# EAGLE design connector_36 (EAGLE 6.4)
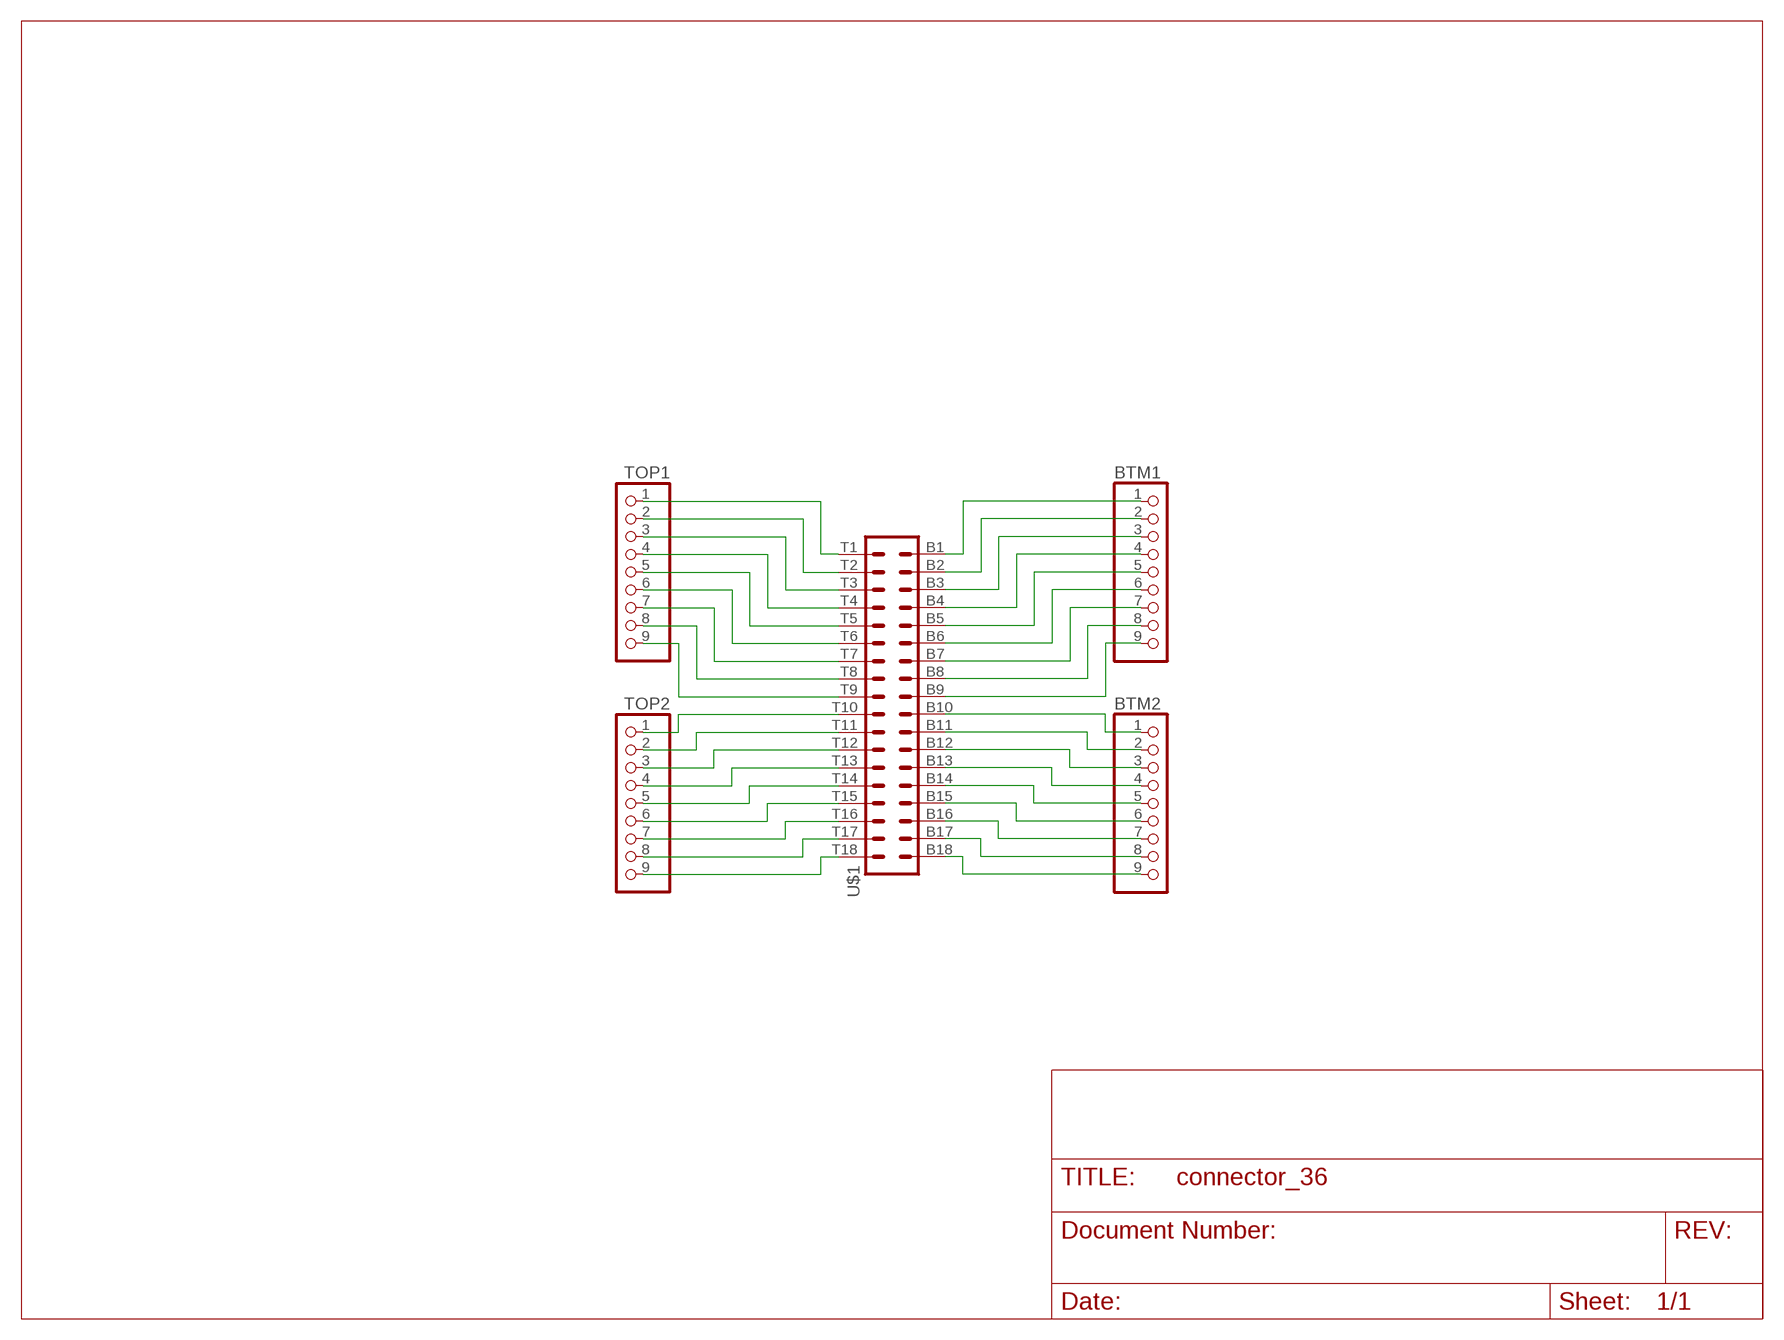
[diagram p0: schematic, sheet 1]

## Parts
BTM1  PINHD-1X9  [1X09]
BTM2  PINHD-1X9  [1X09]
TOP1  PINHD-1X9  [1X09]
TOP2  PINHD-1X9  [1X09]
U$1  OMNETICS_A79024-001  [OMNETICS_A79024-001]

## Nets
N$1: TOP1.1 U$1.T1
N$2: TOP1.2 U$1.T2
N$3: TOP1.3 U$1.T3
N$4: TOP1.4 U$1.T4
N$5: TOP1.5 U$1.T5
N$6: TOP1.6 U$1.T6
N$7: TOP1.7 U$1.T7
N$8: TOP1.8 U$1.T8
N$9: TOP1.9 U$1.T9
N$10: TOP2.1 U$1.T10
N$11: TOP2.2 U$1.T11
N$12: TOP2.3 U$1.T12
N$13: TOP2.4 U$1.T13
N$14: TOP2.5 U$1.T14
N$15: TOP2.6 U$1.T15
N$16: TOP2.7 U$1.T16
N$17: TOP2.8 U$1.T17
N$18: TOP2.9 U$1.T18
N$19: BTM1.1 U$1.B1
N$20: BTM1.2 U$1.B2
N$21: BTM1.3 U$1.B3
N$22: BTM1.4 U$1.B4
N$23: BTM1.5 U$1.B5
N$24: BTM1.6 U$1.B6
N$25: BTM1.7 U$1.B7
N$26: BTM1.8 U$1.B8
N$27: BTM1.9 U$1.B9
N$28: BTM2.1 U$1.B10
N$29: BTM2.2 U$1.B11
N$30: BTM2.3 U$1.B12
N$31: BTM2.4 U$1.B13
N$32: BTM2.5 U$1.B14
N$33: BTM2.6 U$1.B15
N$34: BTM2.7 U$1.B16
N$35: BTM2.8 U$1.B17
N$36: BTM2.9 U$1.B18

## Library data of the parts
BTM1 BTM2 TOP1 TOP2 = pinhead:PINHD-1X9: PIN HEADER
U$1 = omnetics_vic:OMNETICS_A79024-001

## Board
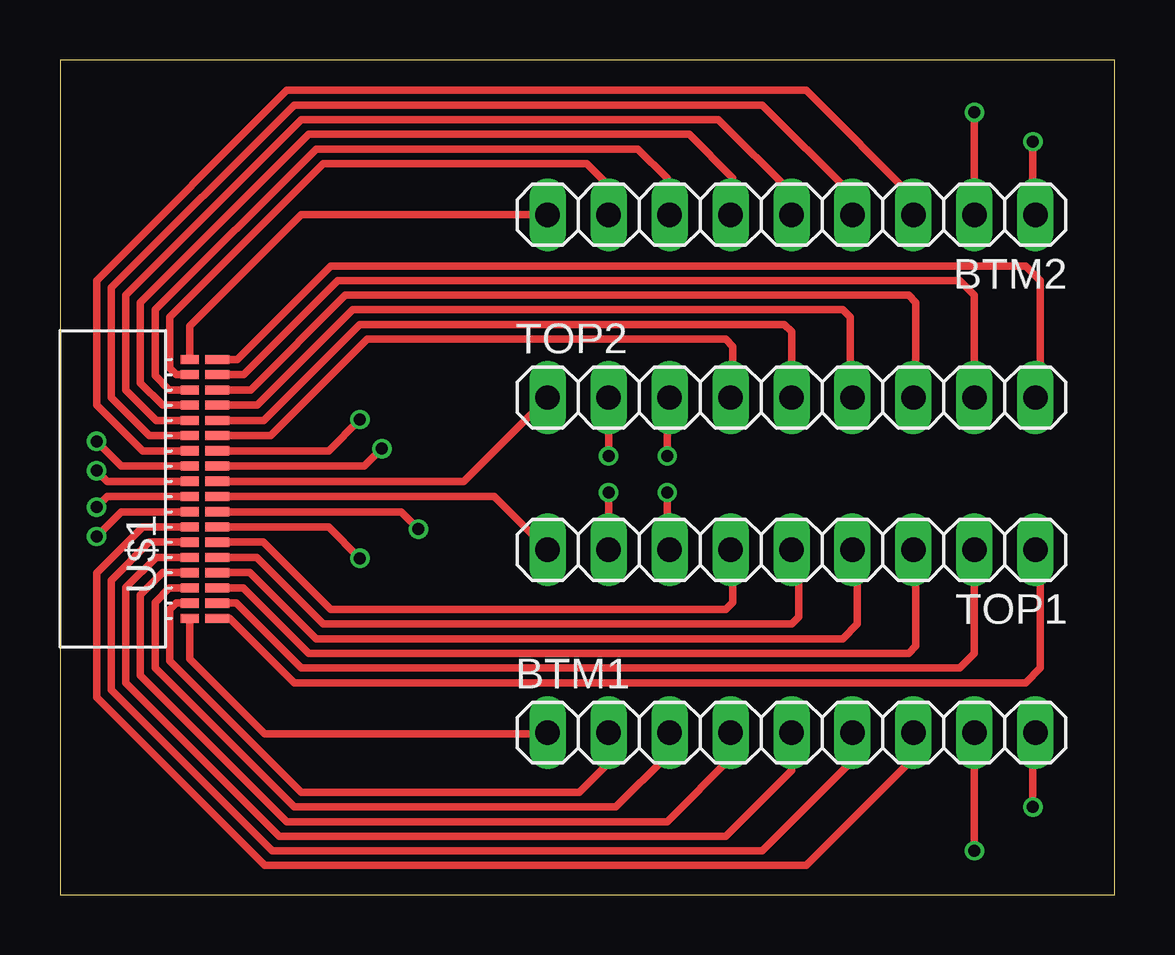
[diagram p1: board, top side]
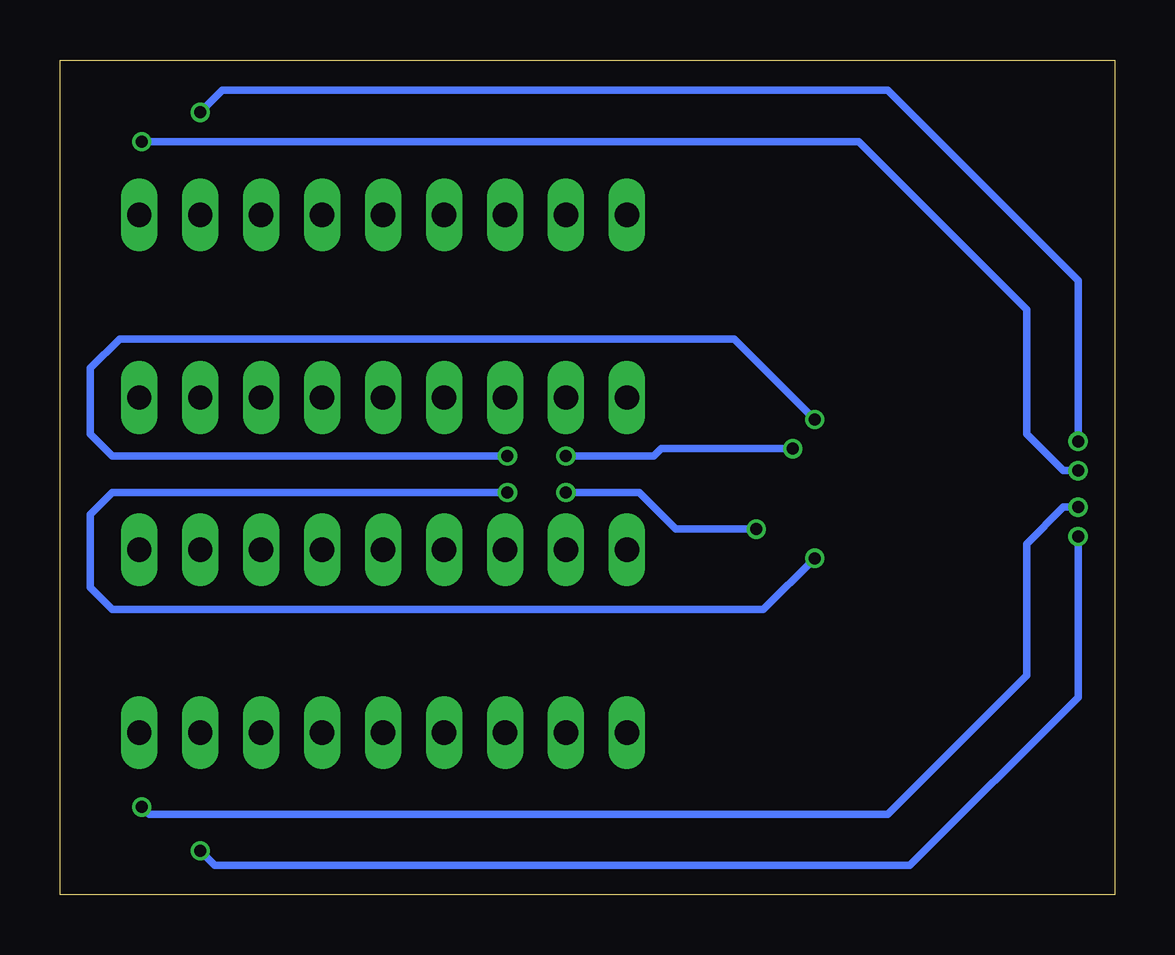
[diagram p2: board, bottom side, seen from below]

Size 43.94 x 34.8 mm. Coordinates in mm from the lower left corner, seen from the top.
Outline: 0,0 43.94,0 43.94,34.8 0,34.8 0,0
Copper layers (1*16): Top 0.035mm / dielectric 1.5mm / Bottom 0.035mm
Design rules "default *": minimum track width 10mil, minimum drill 24mil, track to track 8mil, track to pad 8mil, pad to pad 8mil, via to via 8mil, smd to smd 8mil, copper to edge 40mil, drill to drill 8mil, minimum pad ring 10mil, minimum via ring 6mil, stop-mask expansion 4mil, vias tented up to drill 12mil, thermal gap 10mil

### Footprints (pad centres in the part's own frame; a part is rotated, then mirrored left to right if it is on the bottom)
1X09 = drill 1.016 long: 1 -10.16,0; 2 -7.62,0; 3 -5.08,0; 4 -2.54,0; 5 0,0; 6 2.54,0; 7 5.08,0; 8 7.62,0; 9 10.16,0
OMNETICS_A79024-001 = smd 0.381 x 0.762: B1 -5.397,-0.933; B2 -4.763,-0.933; B3 -4.128,-0.933; B4 -3.493,-0.933; B5 -2.857,-0.933; B6 -2.223,-0.933; B7 -1.587,-0.933; B8 -0.953,-0.933; B9 -0.318,-0.933; B10 0.318,-0.933; B11 0.953,-0.933; B12 1.587,-0.933; B13 2.223,-0.933; B14 2.857,-0.933; B15 3.493,-0.933; B16 4.128,-0.933; B17 4.763,-0.933; B18 5.397,-0.933 | smd 0.381 x 1.016: T1 -5.397,-2.076; T2 -4.763,-2.076; T3 -4.128,-2.076; T4 -3.493,-2.076; T5 -2.857,-2.076; T6 -2.223,-2.076; T7 -1.587,-2.076; T8 -0.953,-2.076; T9 -0.318,-2.076; T10 0.318,-2.076; T11 0.953,-2.076; T12 1.587,-2.076; T13 2.223,-2.076; T14 2.857,-2.076; T15 3.493,-2.076; T16 4.128,-2.076; T17 4.763,-2.076; T18 5.397,-2.076

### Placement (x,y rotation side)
BTM1  30.48,6.76 0 top
BTM2  30.48,28.35 180 top
TOP1  30.48,14.38 180 top
TOP2  30.48,20.73 0 top
U$1  4.48,16.92 90 top

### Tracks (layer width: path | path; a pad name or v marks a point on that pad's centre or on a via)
N$1
  Top 0.305: TOP1.1 40.84,14.17 40.84,9.45 40.23,8.84 9.75,8.84 7.07,11.52 U$1.T1
N$2
  Top 0.305: U$1.T2 7.35,12.15 10.06,9.45 37.49,9.45 38.1,10.06 TOP1.2
N$3
  Top 0.305: TOP1.3 35.66,14.28 35.66,10.36 35.36,10.06 10.36,10.06 7.63,12.79 U$1.T3
N$4
  Top 0.305: U$1.T4 7.91,13.42 10.67,10.67 32.61,10.67 33.22,11.28 33.22,14.17 TOP1.4
N$5
  Top 0.305: U$1.T5 8.19,14.06 10.97,11.28 30.48,11.28 30.79,11.58 30.79,14.07 TOP1.5
N$6
  Top 0.305: TOP1.6 28.04,14.28 28.04,12.19 27.74,11.89 11.28,11.89 8.47,14.69 U$1.T6
N$7  (via drill 0.5 pad 0.3)
  Top 0.305: U$1.T7 11.19,15.33 v12.5,14.02 | TOP1.7 25.3,14.38 v25.3,16.76
  Bottom 0.305: v25.3,16.76 41.76,16.76 42.67,15.85 42.67,12.8 41.76,11.89 14.63,11.89 v12.5,14.02
N$8  (via drill 0.5 pad 0.3)
  Top 0.305: U$1.T8 14.21,15.96 v14.94,15.24 | v22.86,16.76 TOP1.8
  Bottom 0.305: v14.94,15.24 18.29,15.24 19.81,16.76 v22.86,16.76
N$9
  Top 0.305: U$1.T9 18.1,16.6 TOP1.9
N$10
  Top 0.305: U$1.T10 16.83,17.23 TOP2.1
N$11  (via drill 0.5 pad 0.3)
  Top 0.305: TOP2.2 v22.86,18.29 | U$1.T11 12.69,17.87 v13.41,18.59
  Bottom 0.305: v13.41,18.59 18.9,18.59 19.2,18.29 v22.86,18.29
N$12  (via drill 0.5 pad 0.3)
  Top 0.305: TOP2.3 25.3,20.73 v25.3,18.29 | U$1.T12 11.19,18.5 v12.5,19.81
  Bottom 0.305: v12.5,19.81 15.85,23.16 41.45,23.16 42.67,21.95 42.67,19.2 41.76,18.29 v25.3,18.29
N$13
  Top 0.305: U$1.T13 8.78,19.14 12.8,23.16 27.74,23.16 28.04,22.86 28.04,20.83 TOP2.4
N$14
  Top 0.305: U$1.T14 8.5,19.77 12.5,23.77 30.18,23.77 30.48,23.47 TOP2.5
N$15
  Top 0.305: U$1.T15 8.22,20.41 12.19,24.38 32.61,24.38 32.92,24.08 32.92,20.83 TOP2.6
N$16
  Top 0.305: U$1.T16 7.94,21.04 11.89,24.99 35.36,24.99 35.66,24.69 35.66,20.83 TOP2.7
N$17
  Top 0.305: U$1.T17 7.66,21.68 11.58,25.6 37.49,25.6 38.1,24.99 TOP2.8
N$18
  Top 0.305: U$1.T18 7.38,22.31 11.28,26.21 40.23,26.21 40.84,25.6 40.84,20.93 TOP2.9
N$19
  Top 0.305: U$1.B1 5.41,9.83 8.53,6.71 20.27,6.71 BTM1.1
N$20
  Top 0.305: BTM1.2 22.86,5.49 21.64,4.27 10.06,4.27 4.57,9.75 4.57,11.89 4.84,12.15 U$1.B2
N$21
  Top 0.305: U$1.B3 4.56,12.79 3.96,12.19 3.96,9.45 9.75,3.66 23.16,3.66 25.3,5.79 25.3,6.66 BTM1.3
N$22
  Top 0.305: U$1.B4 4.28,13.42 3.35,12.5 3.35,9.14 9.45,3.05 25.3,3.05 28.04,5.79 28.04,6.66 BTM1.4
N$23
  Top 0.305: U$1.B5 4,14.06 2.74,12.8 2.74,8.84 9.14,2.44 27.74,2.44 30.48,5.18 BTM1.5
N$24
  Top 0.305: U$1.B6 3.72,14.69 2.13,13.11 2.13,8.53 8.84,1.83 29.26,1.83 33.22,5.79 33.22,6.55 BTM1.6
N$25
  Top 0.305: U$1.B7 3.44,15.33 1.52,13.41 1.52,8.23 8.53,1.22 31.09,1.22 35.66,5.79 35.66,6.66 BTM1.7
N$26  (via drill 0.5 pad 0.3)
  Top 0.305: U$1.B8 2.55,15.96 v1.52,14.94 | v38.1,1.83 BTM1.8
  Bottom 0.305: v1.52,14.94 1.52,8.23 8.53,1.22 37.49,1.22 v38.1,1.83
N$27  (via drill 0.5 pad 0.3)
  Top 0.305: U$1.B9 1.97,16.6 v1.52,16.15 | v40.54,3.66 40.54,6.66 BTM1.9
  Bottom 0.305: v1.52,16.15 2.13,16.15 3.66,14.63 3.66,9.14 9.45,3.35 40.23,3.35 v40.54,3.66
N$28  (via drill 0.5 pad 0.3)
  Top 0.305: U$1.B10 1.97,17.23 v1.52,17.68 | v40.54,31.39 40.54,28.45 BTM2.1
  Bottom 0.305: v1.52,17.68 2.13,17.68 3.66,19.2 3.66,24.38 10.67,31.39 v40.54,31.39
N$29  (via drill 0.5 pad 0.3)
  Top 0.305: U$1.B11 2.55,17.87 v1.52,18.9 | v38.1,32.61 BTM2.2
  Bottom 0.305: v1.52,18.9 1.52,25.6 9.45,33.53 37.19,33.53 v38.1,32.61
N$30
  Top 0.305: U$1.B12 3.44,18.5 1.52,20.42 1.52,25.6 9.45,33.53 31.09,33.53 35.66,28.96 35.66,28.45 BTM2.3
N$31
  Top 0.305: U$1.B13 3.72,19.14 2.13,20.73 2.13,25.3 9.75,32.92 29.26,32.92 32.92,29.26 32.92,28.45 BTM2.4
N$32
  Top 0.305: U$1.B14 4,19.77 2.74,21.03 2.74,24.99 10.06,32.31 27.43,32.31 30.48,29.26 BTM2.5
N$33
  Top 0.305: U$1.B15 4.28,20.41 3.35,21.34 3.35,24.69 10.36,31.7 26.21,31.7 28.04,29.87 28.04,28.45 BTM2.6
N$34
  Top 0.305: U$1.B16 4.56,21.04 3.96,21.64 3.96,24.38 10.67,31.09 24.08,31.09 25.3,29.87 25.3,28.45 BTM2.7
N$35
  Top 0.305: U$1.B17 4.84,21.68 4.57,21.95 4.57,24.08 10.97,30.48 21.95,30.48 22.86,29.57 BTM2.8
N$36
  Top 0.305: U$1.B18 5.41,23.7 10.06,28.35 BTM2.9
